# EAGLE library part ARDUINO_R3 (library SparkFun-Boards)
Arduino R3 Footprint with SPI header Arduino Uno R3 Compatible Footprint. Matches PCB size of the original board. SparkFun Products: SAMD21 Dev Breakout RedBoard
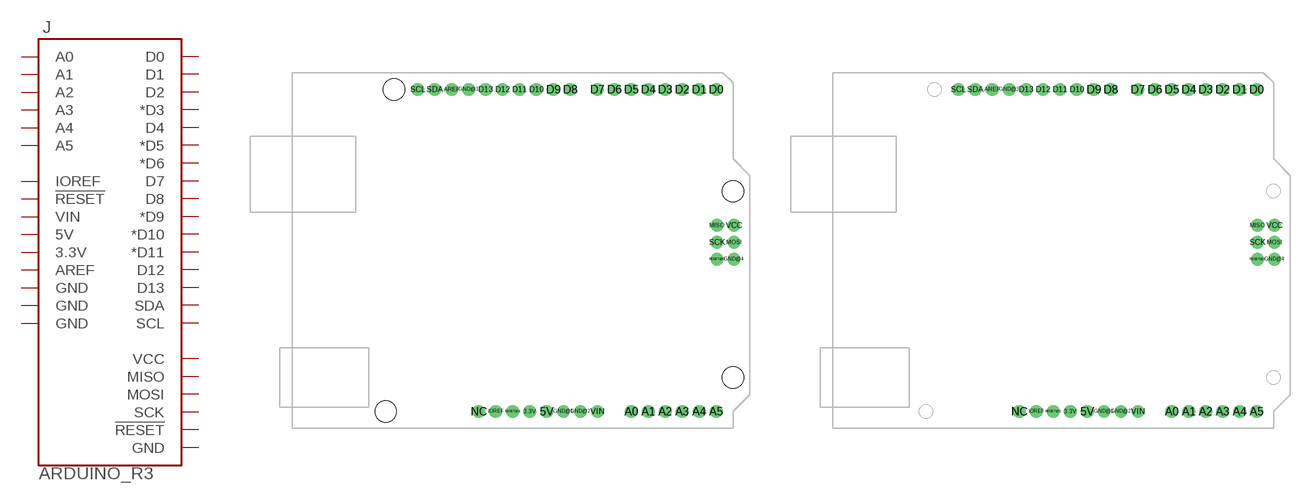
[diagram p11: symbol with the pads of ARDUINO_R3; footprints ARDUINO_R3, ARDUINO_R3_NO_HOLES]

Designator prefix J

## ARDUINO_R3  [ARDUINO_R3]
3.3V  3.3V
5V  5V
A0  A0
A1  A1
A2  A2
A3  A3
A4  A4
A5  A5
AREF  AREF
D0  D0
D1  D1
D2  D2
D3  *D3
D4  D4
D5  *D5
D6  *D6
D7  D7
D8  D8
D9  *D9
D10  *D10
D11  *D11
D12  D12
D13  D13
GND@1  GND
GND@2  GND
GND@3  GND
GND@4  GND
IOREF  IOREF
MISO  MISO
MOSI  MOSI
RESET@1  !RESET!
RESET@2  !RESET!
SCK  SCK
SCL  SCL
SDA  SDA
VCC  VCC
VIN  VIN

## ARDUINO_R3NO_HOLES  [ARDUINO_R3_NO_HOLES]
Pads as for ARDUINO_R3

## Footprint ARDUINO_R3 (pad centres in mm)
Arduino Uno Footprint R3
drill 1.016 pad 1.93: 3.3V 35.56,2.54; 5V 38.1,2.54; A0 50.8,2.54; A1 53.34,2.54; A2 55.88,2.54; A3 58.42,2.54; A4 60.96,2.54; A5 63.5,2.54; AREF 23.876,50.8; D0 63.5,50.8; D1 60.96,50.8; D2 58.42,50.8; D3 55.88,50.8; D4 53.34,50.8; D5 50.8,50.8; D6 48.26,50.8; D7 45.72,50.8; D8 41.656,50.8; D9 39.116,50.8; D10 36.576,50.8; D11 34.036,50.8; D12 31.496,50.8; D13 28.956,50.8; GND@1 40.64,2.54; GND@2 43.18,2.54; GND@3 26.416,50.8; GND@4 66.18,25.35; IOREF 30.48,2.54; MISO 63.64,30.43; MOSI 66.18,27.89; NC 27.94,2.54; RESET@1 33.02,2.54; RESET@2 63.64,25.35; SCK 63.64,27.89; SCL 18.796,50.8; SDA 21.336,50.8; VCC 66.18,30.43; VIN 45.72,2.54
hole 3.175 at 15.24,50.8
hole 3.175 at 66.04,35.56
hole 3.175 at 66.04,7.62
hole 3.175 at 13.97,2.54

## Footprint ARDUINO_R3_NO_HOLES (pad centres in mm)
drill 1.016 pad 1.93: 3.3V 35.56,2.54; 5V 38.1,2.54; A0 50.8,2.54; A1 53.34,2.54; A2 55.88,2.54; A3 58.42,2.54; A4 60.96,2.54; A5 63.5,2.54; AREF 23.876,50.8; D0 63.5,50.8; D1 60.96,50.8; D2 58.42,50.8; D3 55.88,50.8; D4 53.34,50.8; D5 50.8,50.8; D6 48.26,50.8; D7 45.72,50.8; D8 41.656,50.8; D9 39.116,50.8; D10 36.576,50.8; D11 34.036,50.8; D12 31.496,50.8; D13 28.956,50.8; GND@1 40.64,2.54; GND@2 43.18,2.54; GND@3 26.416,50.8; GND@4 66.18,25.35; IOREF 30.48,2.54; MISO 63.64,30.43; MOSI 66.18,27.89; NC 27.94,2.54; RESET@1 33.02,2.54; RESET@2 63.64,25.35; SCK 63.64,27.89; SCL 18.796,50.8; SDA 21.336,50.8; VCC 66.18,30.43; VIN 45.72,2.54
